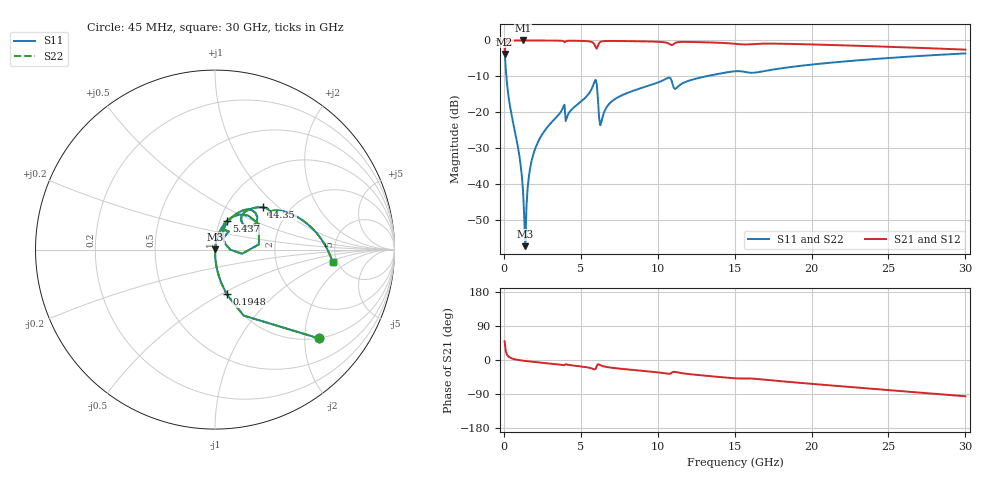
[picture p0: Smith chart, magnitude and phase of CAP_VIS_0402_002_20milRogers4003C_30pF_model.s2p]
! S-parameter model data by Modelithics Inc.  support@modelithics.com  813-866-6335  Tampa FL USA
! S-Parameter data specifications:
! Substrate: 20-mil Rogers 4003C, substrate thickness, H=0.508mm, Dielectric constant, Er=3.75
! PCB Mounting Pad Footprint: Pad width, PadW=0.50mm , Pad length, PadL=0.50mm , Pad gap, PadG (edge-to-edge)=0.40mm , Reference planes=1.4mm apart
! Created Wed Nov 18 12:53:48 2015
# hz S ma R 50
! 2 Port Network Data from SP1.SP block
! freq  magS11  angS11  magS21  angS21  magS12  angS12  magS22  angS22
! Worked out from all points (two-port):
!   401 points, 45 MHz to 30 GHz, reference 50 ohm
!   highest |S21| = -0.01 dB at 1.243 GHz (marker M1); lowest = -3.8 dB at 45 MHz (marker M2)
!   |S21| within 3 dB of the highest: 63.7 MHz to end of sweep
!   lowest |S11| = -57.3 dB at 1.393 GHz (marker M3), VSWR 1.00, Z = 50.1 + j0.0797 ohm
!   |S11| at or under -10 dB: 159.7 MHz to 13.14 GHz (12.98 GHz wide, 195 % of centre)
!   |S22| runs from -57.3 to -2.4 dB; largest |S21 - S12| = 0
!   S11 on the Smith chart (normalised r, x): 45 MHz: 1.00, -2.34; 194.8 MHz: 1.00, -0.53; 5.437 GHz: 1.08, +0.35; 14.35 GHz: 1.47, +0.79; 30 GHz: 4.57, -1.16
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4.5e7  0.7608 -40.5  0.6489 49.5  0.6489 49.5  0.7608 -40.5
1.94775e8  0.2568 -75.4  0.966 14.5  0.966 14.5  0.2568 -75.4
3.4455e8  0.1422 -82.2  0.9893 7.6  0.9893 7.6  0.1422 -82.2
1.018538e9  0.02359 -88.2  0.9988 -0.4  0.9988 -0.4  0.02359 -88.2
1.2432e9  0.007997 -84.4  0.9989 -1.7  0.9989 -1.7  0.007997 -84.4
1.392975e9  0.001366 35.6  0.9989 -2.5  0.9989 -2.5  0.001366 35.6
1.767412e9  0.01953 82.2  0.9985 -4.2  0.9985 -4.2  0.01953 82.2
2.291625e9  0.04152 81.6  0.9977 -6.4  0.9977 -6.4  0.04152 81.6
3.789375e9  0.1094 73.7  0.9875 -13.0  0.9875 -13.0  0.1094 73.7
4.163812e9  0.09246 73.7  0.9897 -12.6  0.9897 -12.6  0.09246 73.7
5.062462e9  0.144 71.1  0.985 -17.2  0.985 -17.2  0.144 71.1
5.4369e9  0.1725 67.5  0.976 -19.5  0.976 -19.5  0.1725 67.5
5.886225e9  0.2649 45.8  0.8803 -24.8  0.8803 -24.8  0.2649 45.8
6.33555e9  0.07276 48.5  0.9651 -14.9  0.9651 -14.9  0.07276 48.5
7.2342e9  0.1534 66.4  0.9826 -21.6  0.9826 -21.6  0.1534 66.4
1.007992e10  0.2628 55.2  0.9565 -33.0  0.9565 -33.0  0.2628 55.2
1.120324e10  0.2158 46.8  0.9347 -32.0  0.9347 -32.0  0.2158 46.8
1.434851e10  0.3551 41.5  0.9199 -46.1  0.9199 -46.1  0.3551 41.5
1.50225e10  0.3719 37.0  0.8976 -48.3  0.8976 -48.3  0.3719 37.0
2.003996e10  0.4617 26.0  0.8788 -63.1  0.8788 -63.1  0.4617 26.0
2.505742e10  0.5699 9.8  0.815 -79.6  0.815 -79.6  0.5699 9.8
3e10  0.6598 -6.2  0.7445 -95.8  0.7445 -95.8  0.6598 -6.2
